{attribute 'no-analysis'}
FUNCTION_BLOCK FB_SboControl EXTENDS FB_Control
VAR
	_eControlState: E_SboControlState; (*State of control state machine*)
	_fbSboTimer: TON; (*Timer to monitor 'sboTimeout'*)
END_VAR

(*This method is called when Cancel_req is received.
It shall check whether the Cancel request is valid and return FALSE as well as an error code if it is not.*)
METHOD PROTECTED _CheckCancelReq : BOOL
VAR_INPUT
	ipDai: I_AcsiDataAccessInfoClass; (*Additional data access info*)
END_VAR
VAR_OUTPUT
	eError: E_AcsiServiceError; (*Error code for negative response*)
END_VAR
VAR
	ipAA: I_ScsmAssociationClass; (*Interface pointer to application association*)
	stRemoteAddr: ST_SockAddr; (*Address of the client that sent the Cancel_req*)
END_VAR
IF (_ipCtrl <> 0) AND_THEN (_ipCtrl.ipCancel <> 0) THEN
	ScsmAssociation_From_Dai(in:=ipDai, out=>ipAA);
	(* Don't allow control if 'ctlModel' is set to 'status-only' *)
	IF (_ipCtrl.ipCtlModel <> 0) AND_THEN (_ipCtrl.ipCtlModel.eValue = E_AcsiCtlModels.StatusOnly) THEN
		_SendLastApplError(ipAA:=ipAA, ipCtrlData:=_ipCtrl.ipCancel, eError:=E_AcsiApplError.NoError, ipOrigin:=_ipCtrl.ipCancel.ipOrigin, ipCtlNum:=_ipCtrl.ipCancel.ipCtlNum, eAddCause:=E_AcsiApplAddCause.Unknown);
		RETURN;
	(* Cancel is always allowed in state 'Unselected' *)
	ELSIF (_eControlState = E_SboControlState.Unselected) THEN
		_CheckCancelReq:=TRUE;
		RETURN;
	(* Cancel is only allowed by the same client that sent the last accepted Sel_req *)
	ELSIF (RemoteAddress_From_ScsmAssociation(in:=ipAA, out=>stRemoteAddr)) AND_THEN (stRemoteAddr.sAddr <> _stCurrrentIp.sAddr) THEN
		_SendLastApplError(ipAA:=ipAA, ipCtrlData:=_ipCtrl.ipCancel, eError:=E_AcsiApplError.NoError, ipOrigin:=_ipCtrl.ipCancel.ipOrigin, ipCtlNum:=_ipCtrl.ipCancel.ipCtlNum, eAddCause:=E_AcsiApplAddCause.LockedByOtherClient);
		RETURN;
	(* Cancel is not allowed in state 'Operate' *)
	ELSIF (_eControlState = E_SboControlState.Operate) THEN
		_SendLastApplError(ipAA:=ipAA, ipCtrlData:=_ipCtrl.ipCancel, eError:=E_AcsiApplError.NoError, ipOrigin:=_ipCtrl.ipCancel.ipOrigin, ipCtlNum:=_ipCtrl.ipCancel.ipCtlNum, eAddCause:=E_AcsiApplAddCause.CommandAlreadyInExecution);
		RETURN;
	(* Cancel is valid *)
	ELSE
		_CheckCancelReq:=TRUE;
	END_IF
END_IF
END_METHOD

//Resets all local values
METHOD PROTECTED _Reset
VAR
END_VAR
SUPER^._Reset();
(* Reset timer *)
_fbSboTimer(IN:=FALSE);
END_METHOD

METHOD Execute : BOOL
VAR
	bTestOk: BOOL; (*Used to cache the return value of the last '_OperativeTest' or '_DynamicTest' method call*)
	eError: E_AcsiServiceError; (*Used to cache the returned error of the last '_OperativeTest' or '_DynamicTest' method call*)
	tValue: T_UtcTime; (*Used to cache the current system time for 'tOpOk'*)
END_VAR
IF (_ipCtrl <> 0) AND_THEN (_ipCtrl.ipOper <> 0) THEN
	(* Initialize function block in the first cycle *)
	IF NOT bInit THEN
		_Init();
		bInit:=TRUE;
	END_IF

	CASE _eControlState OF
		E_SboControlState.Unselected:
			(* Check if ControlState changed in the last cycle *)
			IF bNewState THEN
				bNewState:=FALSE;
				_Reset();
				(* Reset 'stSeld' *)
				IF (_ipCtrl.ipStSeld <> 0) THEN
					_ipCtrl.ipStSeld.bValue:=FALSE;
				END_IF
			END_IF
			(* Check if a valid Cancel_req was received *)
			IF bCancelReq THEN
				bCancelReq:=FALSE;
			END_IF
			(* Check if a valid Sel_req was received *)
			IF bSelReq THEN
				bSelReq:=FALSE;
				(* Set 'stSeld' *)
				IF (_ipCtrl.ipStSeld <> 0) THEN
					_ipCtrl.ipStSeld.bValue:=TRUE;
				END_IF
				(* Go to next ControlState *)
				_eControlState:=E_SboControlState.Ready;
				bNewState:=TRUE;
			END_IF

		E_SboControlState.Ready:
			(* Check if ControlState changed in the last cycle *)
			IF bNewState THEN
				bNewState:=FALSE;
				(* Start timer *)
				IF (_ipCtrl.ipSboTimeout <> 0) THEN
					_fbSboTimer(IN:=TRUE, PT:=DWORD_TO_TIME(_ipCtrl.ipSboTimeout.nValue));
				END_IF
			END_IF
			_fbSboTimer();
			(* Check if a valid Cancel_req was received, 'sboTimeout' was exceeded or the association was lost *)
			IF bCancelReq OR_ELSE _fbSboTimer.Q OR_ELSE ((_ipCurrentAA <> 0) AND_THEN (_ipCurrentAA.eState <> E_AsyncEnvironmentState.Established)) THEN
				bCancelReq:=FALSE;
				_fbSboTimer(IN:=FALSE);
				(* Go to next ControlState *)
				_eControlState:=E_SboControlState.EndSelection;
				bNewState:=TRUE;
			END_IF
			(* Check if a valid Oper_req was received *)
			IF bOperReq THEN
				bOperReq:=FALSE;
				(* Go to next ControlState *)
				_eControlState:=E_SboControlState.PerformTest;
				bNewState:=TRUE;
			END_IF

		E_SboControlState.PerformTest:
			(* Check if ControlState changed in the last cycle *)
			IF bNewState THEN
				bNewState:=FALSE;
				(* Set 'opRcvd' *)
				IF (_ipCtrl.ipOpRcvd <> 0) THEN
					_ipCtrl.ipOpRcvd.bValue:=TRUE;
				END_IF
			END_IF
			(* Check if a valid Cancel_req was received *)
			IF bCancelReq THEN
				bCancelReq:=FALSE;
				(* Send Oper_resp- *)
				_SendLastApplError(ipAA:=_ipCurrentAA, ipCtrlData:=_ipCtrl.ipOper, eError:=E_AcsiApplError.NoError, ipOrigin:=_ipCtrl.ipOper.ipOrigin, ipCtlNum:=_ipCtrl.ipOper.ipCtlNum, eAddCause:=E_AcsiApplAddCause.AbortionByCancel);
				fbOperCompletion.SetCompleted();
				fbOperCompletion.eServiceError:=E_AcsiServiceError.AccessViolation;
				(* Go to ControlState 'EndSelection' *)
				_eControlState:=E_SboControlState.EndSelection;
				bNewState:=TRUE;
			END_IF
			(* Trigger the operative test until it is finished *)
			IF _OperativeTest(bOperativeTestOk=>bTestOk, eError=>eError) THEN
				(* Reset 'opRcvd' *)
				IF (_ipCtrl.ipOpRcvd <> 0) THEN
					_ipCtrl.ipOpRcvd.bValue:=FALSE;
				END_IF
				IF bTestOk THEN
					(* Go to next ControlState *)
					_eControlState:=E_SboControlState.WaitForExecution;
				ELSE
					fbOperCompletion.SetCompleted();
					fbOperCompletion.eServiceError:=eError;
					(* Go to ControlState 'EndSelection' *)
					_eControlState:=E_SboControlState.EndSelection;
				END_IF
				bNewState:=TRUE;
			END_IF

		E_SboControlState.WaitForExecution:
			(* Check if ControlState changed in the last cycle *)
			IF bNewState THEN
				bNewState:=FALSE;
			END_IF
			(* Check if a Cancel_req was received *)
			IF bCancelReq THEN
				bCancelReq:=FALSE;
				(* Send Oper_resp- *)
				_SendLastApplError(ipAA:=_ipCurrentAA, ipCtrlData:=_ipCtrl.ipOper, eError:=E_AcsiApplError.NoError, ipOrigin:=_ipCtrl.ipOper.ipOrigin, ipCtlNum:=_ipCtrl.ipOper.ipCtlNum, eAddCause:=E_AcsiApplAddCause.AbortionByCancel);
				fbOperCompletion.SetCompleted();
				fbOperCompletion.eServiceError:=E_AcsiServiceError.AccessViolation;
				(* Go to ControlState 'EndSelection' *)
				_eControlState:=E_SboControlState.EndSelection;
				bNewState:=TRUE;
			END_IF
			(* Trigger the dynamic test until it is finished *)
			IF _DynamicTest(bDynamicTestOk=>bTestOk, eError=>eError) THEN
				fbOperCompletion.SetCompleted();
				IF bTestOk THEN
					(* Go to next ControlState *)
					IF (_ipBehVal <> 0) AND_THEN ((_ipBehVal.eValue = E_AcsiBeh.TestBlocked) OR_ELSE (_ipBehVal.eValue = E_AcsiBeh.OnBlocked)) THEN
						_eControlState:=E_SboControlState.MirrorBlockedCommand;
					ELSE
						_eControlState:=E_SboControlState.Operate;
					END_IF
				ELSE
					fbOperCompletion.eServiceError:=eError;
					(* Go to ControlState 'EndSelection' *)
					_eControlState:=E_SboControlState.EndSelection;
				END_IF
				bNewState:=TRUE;
			END_IF

		E_SboControlState.Operate:
			(* Check if ControlState changed in the last cycle *)
			IF bNewState THEN
				bNewState:=FALSE;
				(* Set 'opOk' *)
				IF (_ipCtrl.ipOpOk <> 0) THEN
					_ipCtrl.ipOpOk.bValue:=TRUE;
				END_IF
				(* Set 'tOpOk' *)
				IF (_ipCtrl.ipTOpOk <> 0) AND_THEN (_ipCurrentAA <> 0) AND_THEN (_ipCurrentAA.GetSystemTime(tT=>tValue)) THEN
					_ipCtrl.ipTOpOk.tValue:=tValue;
				END_IF
			END_IF
			(* Update value *)
			_SetValue(uCtlVal:=_ipCtrl.ipOper.uCtlVal, ipCtlVal_AV:=_ipCtrl.ipOper.ipCtlVal_AnalogueValue);
			(* Update Timestamp 't' *)
			_UpdateTimestampValue(ipAA:=_ipCurrentAA);

			(* Reset 'opOk' *)
			IF (_ipCtrl.ipOpOk <> 0) THEN
				_ipCtrl.ipOpOk.bValue:=FALSE;
			END_IF
			(* Go to next ControlState *)
			IF (_ipCtrl.ipSboClass <> 0) AND_THEN (_ipCtrl.ipSboClass.eValue = E_AcsiSboClasses.OperateMany) THEN
				_eControlState:=E_SboControlState.Ready;
			ELSE
				_eControlState:=E_SboControlState.EndSelection;
			END_IF
			bNewState:=TRUE;

		E_SboControlState.MirrorBlockedCommand:
			(* Check if ControlState changed in the last cycle *)
			IF bNewState THEN
				bNewState:=FALSE;
				(* Set 'opOk' *)
				IF (_ipCtrl.ipOpOk <> 0) THEN
					_ipCtrl.ipOpOk.bValue:=TRUE;
				END_IF
				(* Set 'tOpOk' *)
				IF (_ipCtrl.ipTOpOk <> 0) AND_THEN (_ipCurrentAA <> 0) AND_THEN (_ipCurrentAA.GetSystemTime(tT=>tValue)) THEN
					_ipCtrl.ipTOpOk.tValue:=tValue;
				END_IF
			END_IF
			(* Reset 'opOk' *)
			IF (_ipCtrl.ipOpOk <> 0) THEN
				_ipCtrl.ipOpOk.bValue:=FALSE;
			END_IF
			(* Go to next ControlState *)
			IF (_ipCtrl.ipSboClass <> 0) AND_THEN (_ipCtrl.ipSboClass.eValue = E_AcsiSboClasses.OperateMany) THEN
				_eControlState:=E_SboControlState.Ready;
			ELSE
				_eControlState:=E_SboControlState.EndSelection;
			END_IF
			bNewState:=TRUE;

		E_SboControlState.EndSelection:
			(* Check if ControlState changed in the last cycle *)
			IF bNewState THEN
				bNewState:=FALSE;
				(* Reset 'stSeld' *)
				IF (_ipCtrl.ipStSeld <> 0) THEN
					_ipCtrl.ipStSeld.bValue:=FALSE;
				END_IF
			END_IF
			(* Go to next ControlState *)
			_eControlState:=E_SboControlState.Unselected;
			bNewState:=TRUE;
	END_CASE
END_IF

(* Monitor transmission of LastApplError *)
CASE _nLastApplErrorReqState OF
	0:	RETURN;
	1:
		IF (_ipLastApplErrorReq <> 0) THEN
			Execute:=_ipLastApplErrorReq.Execute();
			IF NOT _ipLastApplErrorReq.IsBusy() THEN
				IF _ipLastApplErrorReq.IsCompleted() THEN
					SUPER^.SetCompleted();
				ELSE
					SUPER^.CopyFrom(ipSource:=_ipLastApplErrorReq);
				END_IF
				_nLastApplErrorReqState:=0;
			END_IF
		END_IF
END_CASE
END_METHOD

METHOD OnCompletionWaitEvent : BOOL
VAR_INPUT
	ipDai: I_AcsiDataAccessInfoClass;
	ipData: I_AcsiCommonDataClass;
	eFc: E_AcsiFc;
END_VAR
VAR_OUTPUT
	ipResult: I_AcsiServiceResultClass := fbCompletion;
END_VAR
VAR
	eServiceError: E_AcsiServiceError;
	ipAA: I_ScsmAssociationClass; (*Interface pointer to application association*)
END_VAR
fbCompletion.SetCompleted();
IF (ipDai = 0) OR_ELSE (ipData = 0) THEN
	fbCompletion.eServiceError:=E_AcsiServiceError.AccessViolation;
	RETURN;
END_IF

(* Check if an Operate request is received *)
IF (ipDai.eService = E_AcsiServiceType.SetDataValues) THEN
	IF	(ipData.sObjectName = 'Oper') THEN
		ScsmAssociation_From_Dai(in:=ipDai, out=>_ipCurrentAA);
		fbOperCompletion.SetBusy();
		ipResult:=fbOperCompletion;
		bOperReq:=TRUE;
		OnCompletionWaitEvent:=TRUE;
	ELSIF (ipData.sObjectName = 'Cancel') THEN
		fbCancelCompletion.SetCompleted();
		ipResult:=fbCancelCompletion;
		IF _CheckCancelReq(ipDai:=ipDai, eError=>eServiceError) THEN
			bCancelReq:=TRUE;
		ELSE
			fbCancelCompletion.eServiceError:=eServiceError;
		END_IF
	END_IF
END_IF
END_METHOD

(*Implementation of user application data update event method.*)
METHOD OnGetVEvent
VAR_INPUT
	ipDai: I_AcsiDataAccessInfoClass; (*Additional data access info*)
	ipData: I_AcsiCommonDataClass; (*Interface pointer to data object*)
	eFc: E_AcsiFc; (*Functional constraint*)
END_VAR
VAR
END_VAR
IF (eFc = E_AcsiFc.CO) AND_THEN (_ipCtrl <> 0) AND_THEN (ipDai <> 0) AND_THEN (ipDai.Read) AND_THEN (ipDai.ipAccessData <> 0) THEN
	IF (ipDai.ipAccessData.sObjectName = 'SBO') AND_THEN (_ipCtrl.ipSBO <> 0) THEN
		(* Reset value of 'SBO' *)
		_ipCtrl.ipSBO.sValue:='';
	END_IF
END_IF
END_METHOD

(*Implementation of user application data update event method.*)
METHOD OnGetVPreEvent : E_AcsiServiceError
VAR_INPUT
	ipDai: I_AcsiDataAccessInfoClass; (*Additional data access info*)
	ipData: I_AcsiCommonDataClass; (*Interface pointer to data object*)
	eFc: E_AcsiFc; (*Functional constraint*)
END_VAR
VAR
END_VAR
IF (eFc = E_AcsiFc.CO) AND_THEN (_ipCtrl <> 0) AND_THEN (ipDai <> 0) AND_THEN (ipDai.Read) AND_THEN (ipDai.ipAccessData <> 0) THEN
	IF (ipDai.ipAccessData.sObjectName = 'SBO') AND_THEN (_ipCtrl.ipSBO <> 0) THEN
		(* Only allow 'Select' requests in state 'Unselected' *)
		IF (_eControlState = E_SboControlState.Unselected) THEN
			_ipCtrl.ipSBO.sValue:=_ipCtrl.ipSBO.GetSboReference();
			bSelReq:=TRUE;
		ELSE
			_ipCtrl.ipSBO.sValue:='';
		END_IF
	END_IF
END_IF
END_METHOD

(*Implementation of user application data update event method.*)
METHOD OnSetVPreEvent : E_AcsiServiceError
VAR_INPUT
	ipDai: I_AcsiDataAccessInfoClass; (*Additional data access info*)
	ipMemory: I_AnyMemoryBuffer; (*Interface pointer to buffer containig new value data*)
	ipData: I_AcsiCommonDataClass; (*Interface pointer to data object*)
	eFc: E_AcsiFc; (*Functional constraint*)
END_VAR
VAR_OUTPUT
	ipLastApplError: I_AcsiDATypeLastApplError; (*IF <> 0 => send LastApplError request*)
END_VAR
VAR
	ipAA: I_ScsmAssociationClass; (*Interface pointer to application association*)
	bItself: BOOL; (*If TRUE => Checking object is sub-data object itself*)
END_VAR
IF (eFc = E_AcsiFc.CO) AND_THEN (_ipCtrl <> 0) AND_THEN (ipDai <> 0) AND_THEN (ipDai.Write) AND_THEN (ipDai.ipAccessData <> 0) AND_THEN (ipData <> 0) AND_THEN ScsmAssociation_From_Dai(in:=ipDai, out=>ipAA) THEN
	IF (_ipCtrl.ipOper <> 0) AND_THEN (_ipCtrl.ipOper.ipOrigin <> 0) AND_THEN (_ipCtrl.ipOper.ipCtlNum <> 0) THEN
		(* Check for invalid write attemps to prevent 'Oper' from being overwritten while a control request is being executed *)
		IF (ipDai.ipAccessData.sObjectName = 'Oper') THEN
			(* Only allow 'Oper' requests in state 'Ready' *)
			IF (_eControlState <> E_SboControlState.Ready) THEN
				ipLastApplError:=ipAA.SetAdditionalCauseDiag(ipCtrlData:=_ipCtrl.ipOper, eError:=E_AcsiApplError.NoError, stOrigin:=_ipCtrl.ipOper.ipOrigin.stOrigin, nCtlNum:=_ipCtrl.ipOper.ipCtlNum.nValue, eAddCause:=E_AcsiApplAddCause.CommandAlreadyInExecution);
				OnSetVPreEvent:=E_AcsiServiceError.AccessViolation;
				RETURN;
			END_IF
		ELSIF (_ipCtrl.ipOper.HasDataSubObject(ipData:=ipDai.ipAccessData, bItself=>bItself) AND_THEN (NOT bItself)) THEN
			(* Don't allow write access to subdata of 'Oper'*)
			ipLastApplError:=ipAA.SetAdditionalCauseDiag(ipCtrlData:=_ipCtrl.ipOper, eError:=E_AcsiApplError.NoError, stOrigin:=_ipCtrl.ipOper.ipOrigin.stOrigin, nCtlNum:=_ipCtrl.ipOper.ipCtlNum.nValue, eAddCause:=E_AcsiApplAddCause.NotSupported);
			OnSetVPreEvent:=E_AcsiServiceError.AccessViolation;
			RETURN;
		END_IF
	END_IF
	IF (_ipCtrl.ipCancel <> 0) AND_THEN (_ipCtrl.ipCancel.ipOrigin <> 0) AND_THEN (_ipCtrl.ipCancel.ipCtlNum <> 0) THEN
		IF (ipDai.ipAccessData.sObjectName <> 'Cancel') AND_THEN (_ipCtrl.ipCancel.HasDataSubObject(ipData:=ipDai.ipAccessData)) THEN
			(* Don't allow write access to subdata of 'Cancel'*)
			ipLastApplError:=ipAA.SetAdditionalCauseDiag(ipCtrlData:=_ipCtrl.ipCancel, eError:=E_AcsiApplError.NoError, stOrigin:=_ipCtrl.ipCancel.ipOrigin.stOrigin, nCtlNum:=_ipCtrl.ipCancel.ipCtlNum.nValue, eAddCause:=E_AcsiApplAddCause.NotSupported);
			OnSetVPreEvent:=E_AcsiServiceError.AccessViolation;
			RETURN;
		END_IF
	END_IF
	IF (ipData.sObjectName = 'SBO') THEN
		(* Don't allow write access to 'SBO'*)
		OnSetVPreEvent:=E_AcsiServiceError.AccessViolation;
		RETURN;
	END_IF
END_IF
END_METHOD

END_FUNCTION_BLOCK
